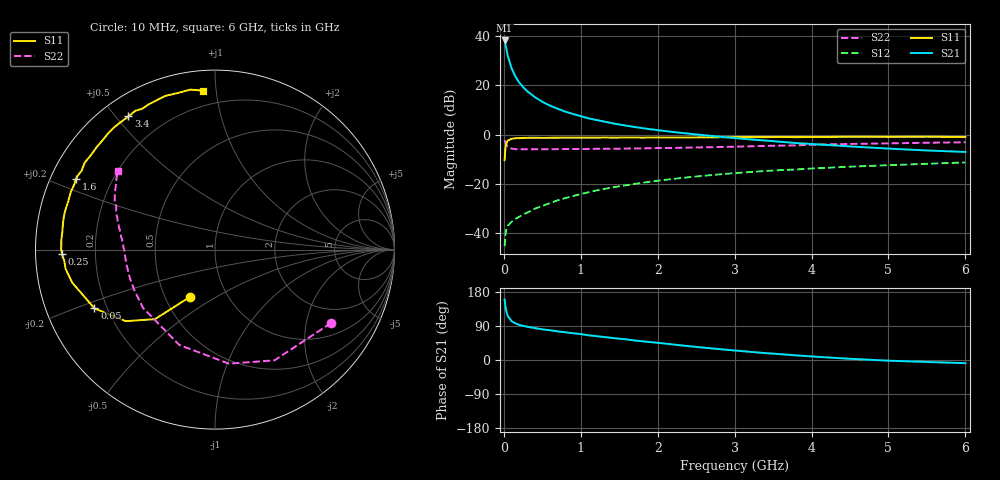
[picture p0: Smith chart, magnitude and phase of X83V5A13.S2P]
! SIEMENS Small Signal Semiconductors
! BFP136W
! Si NPN RF Bipolar Junction Transistor in SOT343
! VCE = 3.5 V  IC = 130 mA
! Common Emitter S-Parameters:  September  1994
# GHz  S  MA  R  50
!  f  S11  S21  S12  S22
! GHz  MAG  ANG  MAG  ANG  MAG  ANG  MAG  ANG
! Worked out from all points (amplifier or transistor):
!   40 points, 10 MHz to 6 GHz, reference 50 ohm
!   highest |S21| = 38.3 dB at 10 MHz (marker M1)
!   |S21| within 3 dB of that: start of sweep to 29.83 MHz
!   unconditionally stable (mu >= 1): 486.3 MHz to 2.913 GHz
!   at 200 MHz: K = 0.73, MSG = 27.4 dB, |S12| = -33.5 dB
!   at 1.5 GHz: K = 1.10, MAG = 10.7 dB, |S12| = -21.1 dB
!   at 6 GHz: K = 0.97, MSG = 2.1 dB, |S12| = -11.4 dB
!   S11 on the Smith chart (normalised r, x): 10 MHz: 0.66, -0.39; 50 MHz: 0.15, -0.23; 250 MHz: 0.08, -0.01; 1.6 GHz: 0.07, +0.24; 3.4 GHz: 0.08, +0.54; 6 GHz: 0.11, +0.92
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0.01  0.3002 -118.1  82.58 159.4  0.0053 68.0  0.7651 -32.3
0.02  0.512 -130.8  69.88 142.3  0.0086 57.4  0.7005 -61.7
0.03  0.6377 -141.3  58.28 130.5  0.0113 48.6  0.6404 -83.0
0.05  0.7471 -154.0  41.04 116.6  0.0138 38.9  0.5673 -110.6
0.1  0.8167 -167.0  22.5 102.7  0.0166 38.2  0.5158 -141.1
0.15  0.8393 -172.7  15.28 96.6  0.0189 41.2  0.5028 -153.4
0.2  0.8416 -175.6  11.47 92.8  0.0211 43.9  0.5001 -160.1
0.25  0.8523 -178.3  9.255 90.0  0.0234 47.4  0.4999 -164.3
0.3  0.8568 179.9  7.734 87.9  0.0254 49.1  0.4988 -167.1
0.4  0.858 176.5  5.827 84.2  0.0306 53.5  0.4999 -171.0
0.5  0.8562 174.0  4.645 81.0  0.035 56.4  0.5007 -173.7
0.6  0.8574 172.0  3.877 78.5  0.0401 58.4  0.5021 -175.4
0.7  0.86 169.6  3.343 75.5  0.0455 60.4  0.5033 -176.7
0.9  0.8624 166.1  2.616 70.5  0.0556 61.2  0.5054 -179.3
1.1  0.8606 161.7  2.14 65.2  0.0664 61.8  0.5084 179.1
1.6  0.8686 153.1  1.507 54.2  0.093 59.9  0.5182 175.0
2.2  0.8688 142.8  1.125 40.9  0.1243 55.4  0.5324 170.4
3.2  0.8835 126.0  0.795 21.6  0.1717 45.8  0.574 161.6
3.4  0.885 123.0  0.753 18.2  0.1809 43.6  0.5863 159.9
4.5  0.9 107.9  0.572 3.2  0.221 33.3  0.6421 150.4
5.5  0.9019 98.8  0.473 -5.2  0.2532 25.6  0.6795 143.8
6  0.8884 94.4  0.441 -8.4  0.2695 21.2  0.6942 141.0
